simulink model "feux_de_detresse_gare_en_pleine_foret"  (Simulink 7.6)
settings: Solver=ode15s  StartTime=0.0  StopTime=100  RelTol=1e-3
InitFcn:
  | clc
  | delete *.mat
libraries: fl_lib x9, elec_lib x8, nesl_utility x3, simulink x1, gaugeslibv2 x1

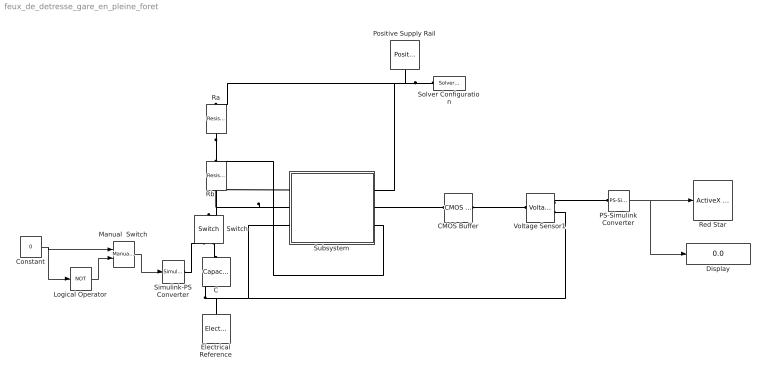
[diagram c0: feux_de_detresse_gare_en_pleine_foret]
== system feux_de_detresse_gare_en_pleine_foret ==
  C : fl_lib/Electrical/Electrical Elements/Capacitor  DialogController=NetworkEngine.DynNeDlgSource  SystemSampleTime=-1  c=1e-3 F  v0=0 V  r=1e-6 Ohm  g=0 1/Ohm  i_Log=off  v_Log=off  vc_Log=off  LocalVarNames=|i|v|vc  LocalVarDescs=|i|v|Internal variable for voltage across capacitor term  LocalVarLogging=[0 0 0]
  CMOS Buffer : elec_lib/Integrated Circuits/Logic/CMOS Buffer  DialogController=NetworkEngine.DynNeDlgSource  SystemSampleTime=-1  V_IL=2 V  V_IH=3 V  C_IN=5 pF  output_type=1  V_OL=0 V  V_OH=5 V  V_CC=5 V  V_meas=5 V  R_OUT=25 Ohm  R_OH=[ 25 250 ] Ohm  I_OH=63 mA  R_OL=[ 30 800 ] Ohm  I_OL=-45 mA  Delay=25 ns  Ron=5 Ohm  Vf=0.6 V  output_state=1  LocalVarLogging=[]
  Constant : Constant  Value=0
  Display : Display
  Electrical Reference : fl_lib/Electrical/Electrical Elements/Electrical Reference  DialogController=NetworkEngine.DynNeDlgSource  SystemSampleTime=-1  i_Log=off  LocalVarNames=|i  LocalVarDescs=|i  LocalVarLogging=0
  Logical Operator : Logic  Operator=NOT  AllPortsSameDT=off  OutDataTypeStr=boolean
  Manual  Switch : simulink/Signal Routing/Manual Switch  SystemSampleTime=-1  sw=0  action=0  varsize=off
  PS-Simulink Converter : nesl_utility/PS-Simulink Converter  DialogController=NetworkEngine.DynNeUtilDlgSource  SystemSampleTime=-1  PhysicalDomain=network_engine_domain  LeftPortType=input  RightPortType=output  SubClassName=ps_output  Unit=1  AffineConversion=off
  Positive Supply Rail : elec_lib/Sources/Positive Supply Rail  DialogController=NetworkEngine.DynNeDlgSource  SystemSampleTime=-1  v0=5 V  current_Log=off  voltage_Log=off  power_Log=off  LocalVarNames=|current|voltage|power  LocalVarDescs=|Current (A)|Voltage (V)|Power (W)  LocalVarLogging=[0 0 0]
  Ra : fl_lib/Electrical/Electrical Elements/Resistor  DialogController=NetworkEngine.DynNeDlgSource  SystemSampleTime=-1  R=1.2 kOhm  i_Log=off  v_Log=off  LocalVarNames=|i|v  LocalVarDescs=|i|v  LocalVarLogging=[0 0]
  Rb : fl_lib/Electrical/Electrical Elements/Resistor  DialogController=NetworkEngine.DynNeDlgSource  SystemSampleTime=-1  R=1.2 kOhm  i_Log=off  v_Log=off  LocalVarNames=|i|v  LocalVarDescs=|i|v  LocalVarLogging=[0 0]
  Red Star : gaugeslibv2/ActiveX Control  progid=MWLED.ledctrl.1  connect=input  input=Value  init=hActx.configuration='LED\Individual\Red Star';hActx.value=1;hActx.Mode=0;hActx.MouseControl=0;  inblock=on  border=on  updateParam=0
  Simulink-PS Converter : nesl_utility/Simulink-PS Converter  DialogController=NetworkEngine.DynNeUtilDlgSource  SystemSampleTime=-1  PhysicalDomain=network_engine_domain  LeftPortType=input  RightPortType=output  SubClassName=ps_input  Unit=1  AffineConversion=off  InputFilterTimeConstant=.001  UdotUserProvided=0
  Solver Configuration : nesl_utility/Solver Configuration  DialogController=NetworkEngine.DynNeUtilDlgSource  SystemSampleTime=-1  PhysicalDomain=network_engine_domain  LeftPortType=input  RightPortType=generic  SubClassName=solver  Accelerate=off  Profile=off  ResidualTolerance=1e-9  MaxNonlinIter=12  MaxModeIter=2  DoFixedCost=off  UseLocalSampling=off  DoDC=off  LinearAlgebra=Sparse  LocalSolverSampleTime=.001  LocalSolverChoice=NE_BACKWARD_EULER_ADVANCER  UseLocalSolver=off
  Subsystem : Subsystem
  Switch : fl_lib/Electrical/Electrical Elements/Switch  DialogController=NetworkEngine.DynNeDlgSource  SystemSampleTime=-1  R_closed=0.01 Ohm  G_open=1e-8 1/Ohm  Threshold=0  i_Log=off  v_Log=off  LocalVarNames=|i|v  LocalVarDescs=|i|v  LocalVarLogging=[0 0]
  Voltage Sensor1 : fl_lib/Electrical/Electrical Sensors/Voltage Sensor  DialogController=NetworkEngine.DynNeDlgSource  SystemSampleTime=-1  i1_Log=off  v1_Log=off  LocalVarNames=|i1|v1  LocalVarDescs=|i1|v1  LocalVarLogging=[]
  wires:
  PS-Simulink Converter/1 -> Red Star/1, Display/1
  Manual  Switch/1 -> Simulink-PS Converter/1
  Logical Operator/1 -> Manual  Switch/2
  Constant/1 -> Manual  Switch/1, Logical Operator/1
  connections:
  Subsystem/LConn1 -- Subsystem/LConn2 -- Rb/LConn1 -- Switch/LConn1
  Voltage Sensor1/RConn2 -- Electrical Reference/LConn1 -- C/RConn1 -- Subsystem/LConn3
  Voltage Sensor1/RConn1 -- PS-Simulink Converter/LConn1
  Solver Configuration/RConn1 -- Ra/RConn1 -- Positive Supply Rail/RConn1 -- Subsystem/RConn1
  Simulink-PS Converter/RConn1 -- Switch/RConn1
  Rb/RConn1 -- Ra/LConn1 -- Subsystem/RConn3
  Switch/RConn2 -- C/LConn1
  Subsystem/RConn2 -- CMOS Buffer/LConn1
  CMOS Buffer/RConn1 -- Voltage Sensor1/LConn1

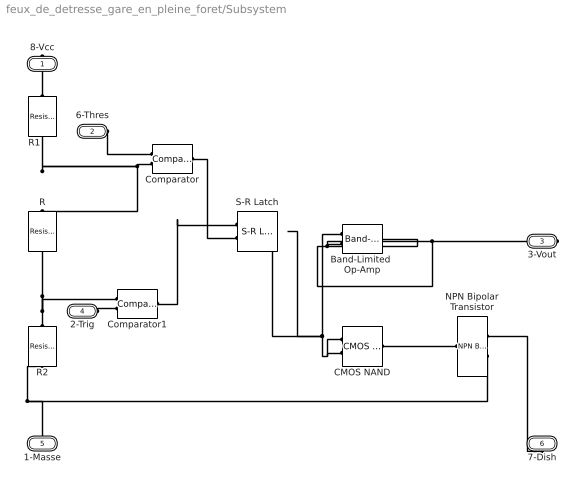
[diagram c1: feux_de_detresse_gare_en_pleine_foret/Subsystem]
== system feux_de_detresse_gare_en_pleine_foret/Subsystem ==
  Band-Limited  Op-Amp : elec_lib/Integrated Circuits/Band-Limited Op-Amp  DialogController=NetworkEngine.DynNeDlgSource  SystemSampleTime=-1  A=1000  Rin=1e+6 Ohm  Rout=100 Ohm  Vmin=-15 V  Vmax=15 V  Vdotmax=1000 V/s  f=1e+5 Hz  V0=0 V  LocalVarLogging=[]
  CMOS NAND : elec_lib/Integrated Circuits/Logic/CMOS NAND  DialogController=NetworkEngine.DynNeDlgSource  SystemSampleTime=-1  V_IL=2 V  V_IH=3 V  C_IN=5 pF  output_type=1  V_OL=0 V  V_OH=5 V  V_CC=5 V  V_meas=5 V  R_OUT=25 Ohm  R_OH=[ 25 250 ] Ohm  I_OH=63 mA  R_OL=[ 30 800 ] Ohm  I_OL=-45 mA  Delay=25 ns  Ron=5 Ohm  Vf=0.6 V  output_state=1  LocalVarLogging=[]
  Comparator : elec_lib/Integrated Circuits/Comparator  DialogController=NetworkEngine.DynNeDlgSource  SystemSampleTime=-1  V_OS=5 mV  V_OL=0 V  V_OH=5 V  C_IN=0 pF  R_OUT=50 Ohm  Delay=0 s  LocalVarLogging=[]
  Comparator1 : elec_lib/Integrated Circuits/Comparator  DialogController=NetworkEngine.DynNeDlgSource  SystemSampleTime=-1  V_OS=5 mV  V_OL=0 V  V_OH=5 V  C_IN=0 pF  R_OUT=50 Ohm  Delay=0 s  LocalVarLogging=[]
  NPN Bipolar Transistor : elec_lib/Semiconductor Devices/NPN Bipolar Transistor  DialogController=NetworkEngine.DynNeDlgSource  SystemSampleTime=-1  parameterization=1  BF=100  IS=1e-14 A  VAF=200 V  hfe=100  hoe=5e-5 1/Ohm  Ic_h=1 mA  V1=0.55 V  I1=0.5 mA  BR=1  Tmeas=25 C  RC=0.01 Ohm  RE=1e-4 Ohm  RB=1 Ohm  C_BC=5 pF  C_BE=5 pF  TF=0 us  TR=0 us  LocalVarLogging=[]
  R : fl_lib/Electrical/Electrical Elements/Resistor  DialogController=NetworkEngine.DynNeDlgSource  SystemSampleTime=-1  R=5 kOhm  i_Log=off  v_Log=off  LocalVarNames=|current|voltage|power  LocalVarDescs=|Resistor current (A)|Voltage across resistor (V)|Power (W)  LocalVarLogging=[0 0 0]
  R1 : fl_lib/Electrical/Electrical Elements/Resistor  DialogController=NetworkEngine.DynNeDlgSource  SystemSampleTime=-1  R=5 kOhm  i_Log=off  v_Log=off  LocalVarNames=|current|voltage|power  LocalVarDescs=|Resistor current (A)|Voltage across resistor (V)|Power (W)  LocalVarLogging=[0 0 0]
  R2 : fl_lib/Electrical/Electrical Elements/Resistor  DialogController=NetworkEngine.DynNeDlgSource  SystemSampleTime=-1  R=5 kOhm  i_Log=off  v_Log=off  LocalVarNames=|current|voltage|power  LocalVarDescs=|Resistor current (A)|Voltage across resistor (V)|Power (W)  LocalVarLogging=[0 0 0]
  S-R Latch : elec_lib/Integrated Circuits/Logic/S-R Latch  DialogController=NetworkEngine.DynNeDlgSource  SystemSampleTime=-1  V_IL=2 V  V_IH=3 V  C_IN=5 pF  output_type=1  V_OL=0 V  V_OH=5 V  V_CC=5 V  V_meas=5 V  R_OUT=25 Ohm  R_OH=[ 25 250 ] Ohm  I_OH=63 mA  R_OL=[ 30 800 ] Ohm  I_OL=-45 mA  Delay=25 ns  Ron=5 Ohm  Vf=0.6 V  output_state=1  LocalVarLogging=[]
  8-Vcc : PMIOPort  Port=1  Side=Right
  6-Thres : PMIOPort  Port=2  Side=Left
  3-Vout : PMIOPort  Port=3  Side=Right
  2-Trig : PMIOPort  Port=4  Side=Left
  1-Masse : PMIOPort  Port=5  Side=Left
  7-Dish : PMIOPort  Port=6  Side=Right
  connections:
  NPN Bipolar Transistor/RConn1 -- 7-Dish/RConn1
  CMOS NAND/RConn1 -- NPN Bipolar Transistor/LConn1
  NPN Bipolar Transistor/RConn2 -- R2/RConn1 -- 1-Masse/RConn1
  2-Trig/RConn1 -- Comparator1/LConn2
  6-Thres/RConn1 -- Comparator/LConn1
  8-Vcc/RConn1 -- R1/LConn1
  Comparator1/RConn1 -- S-R Latch/LConn1
  R2/LConn1 -- R/RConn1 -- Comparator1/LConn1
  Comparator/RConn1 -- S-R Latch/LConn2
  Comparator/LConn2 -- R/LConn1 -- R1/RConn1
  Band-Limited  Op-Amp/LConn2 -- Band-Limited  Op-Amp/RConn1 -- 3-Vout/RConn1
  CMOS NAND/LConn2 -- CMOS NAND/LConn1 -- Band-Limited  Op-Amp/LConn1 -- S-R Latch/RConn1
